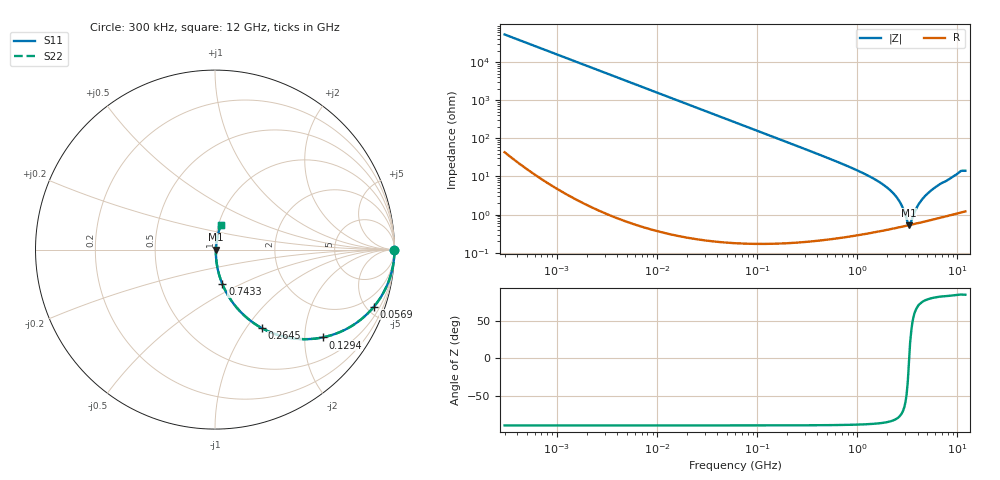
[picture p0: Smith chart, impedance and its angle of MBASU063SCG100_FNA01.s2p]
! MBASU063SCG100_FNA01  S-PARAMETER MODEL  ( Standard Model )
! Model Generated by TAIYO YUDEN Corporation (http://www.ty-top.com)
! Version 1.0
! TAIYO YUDEN Control No. 230609
! Copyright(c) 2023 TAIYO YUDEN CO.,LTD. All Rights Reserved.
! Product Description (link to TY-COMPAS)
! https://ds.yuden.co.jp/TYCOMPAS/or/detail?pn=MBASU063SCG100JFNA01&u=M
! Products Name : Multilayer Ceramic Capacitors
! Characteristics :
!  Capacitance : 10 [pF] , Rated Voltage : 50 [V] , TCC : CG / C0G
!  Case Size : 0.6 x 0.3 / 0.024 x 0.012 [mm/inch] , Thickness : 0.3 / 0.012 [mm/inch]
!  (Conditions: Temperature = 25 [degC] , DC Bias Voltage = 0 [V])
! External Node Assignments :
!  1  o---| |---o  2
! GND o---------o GND
! Frequency Range : 0.3MHz  -  12000MHz  [ 401 STEP ]
# MHZ S RI R 50
! Freq[MHz].  S11 Real  S11 Imag  S21 Real  S21 Imag  S12 Real  S12 Imag  S22 Real  S22 Imag
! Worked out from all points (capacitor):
!   401 points, 300 kHz to 12 GHz, reference 50 ohm
!   read as one part in series: C = 10 pF near 316.3 kHz
!   lowest |Z| = 530 mohm at 3.277 GHz (marker M1)
!   series resonance near 3.294 GHz, so ESL is about 230 pH
!   S11 on the Smith chart (normalised r, x): 300 kHz: open; 56.9 MHz: 1.00, -5.57; 129.4 MHz: 1.00, -2.45; 264.5 MHz: 1.00, -1.19; 743.3 MHz: 1.01, -0.41; 12 GHz: 1.02, +0.28
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0.3  1 -0.00189  5.12e-06 0.00189  5.12e-06 0.00189  1 -0.00189
1.769972  0.9999 -0.0112  0.000127 0.0112  0.000127 0.0112  0.9999 -0.0112
10.44266  0.9957 -0.0655  0.00433 0.0655  0.00433 0.0655  0.9957 -0.0655
25.70316  0.9744 -0.1579  0.0256 0.1579  0.0256 0.1579  0.9744 -0.1579
56.90376  0.8858 -0.3178  0.1142 0.3178  0.1142 0.3178  0.8858 -0.3178
60  0.8746 -0.3308  0.1254 0.3308  0.1254 0.3308  0.8746 -0.3308
129.3602  0.5997 -0.4893  0.4003 0.4893  0.4003 0.4893  0.5997 -0.4893
264.5085  0.2627 -0.4385  0.7373 0.4385  0.7373 0.4385  0.2627 -0.4385
353.9943  0.1651 -0.3691  0.8349 0.3691  0.8349 0.3691  0.1651 -0.3691
743.2595  0.0417 -0.1936  0.9583 0.1936  0.9583 0.1936  0.0417 -0.1936
1403.667  0.0117 -0.0911  0.9883 0.0911  0.9883 0.0911  0.0117 -0.0911
2088.533  0.00612 -0.045  0.9939 0.045  0.9939 0.045  0.00612 -0.045
2650.866  0.00509 -0.021  0.9949 0.021  0.9949 0.021  0.00509 -0.021
2870.14  0.00504 -0.0133  0.995 0.0133  0.995 0.0133  0.00504 -0.0133
3107.553  0.00512 -0.00565  0.9949 0.00565  0.9949 0.00565  0.00512 -0.00565
3276.641  0.00525 -0.000485  0.9947 0.000485  0.9947 0.000485  0.00525 -0.000485
3454.93  0.00543 0.00397  0.9946 -0.00397  0.9946 -0.00397  0.00543 0.00397
4158.869  0.00641 0.0188  0.9936 -0.0188  0.9936 -0.0188  0.00641 0.0188
5006.236  0.00796 0.0341  0.992 -0.0341  0.992 -0.0341  0.00796 0.0341
6354.153  0.0111 0.0561  0.9889 -0.0561  0.9889 -0.0561  0.0111 0.0561
10511.28  0.0273 0.1258  0.9727 -0.1258  0.9727 -0.1258  0.0273 0.1258
12000  0.0308 0.1349  0.9692 -0.1349  0.9692 -0.1349  0.0308 0.1349
